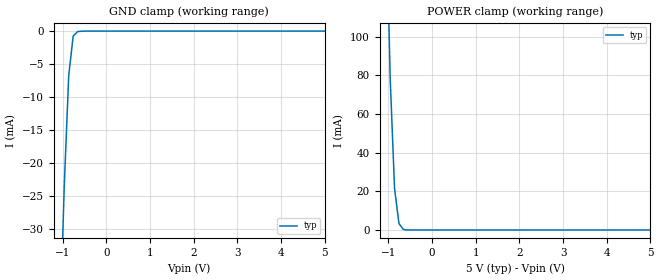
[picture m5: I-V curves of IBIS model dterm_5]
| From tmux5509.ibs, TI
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| dterm_5
[Model]   dterm_5
Model_type   Terminator
|   typ   min   max
C_comp   6.362683e-12   NA   NA
[Voltage Range]   5   NA   NA
[Temperature Range]   27   NA   NA
[Power Clamp Reference]   5   NA   NA
[GND Clamp Reference]   0   NA   NA
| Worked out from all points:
|   GND clamp passes 1 mA (typ) near -0.76 V on its own axis
|   POWER clamp passes 1 mA (typ) near -0.68 V on its own axis
[GND Clamp]
|   Voltage   I(typ)   I(min)   I(max)
-5V       -2.839A    NA         NA
-1.061V   -45mA      NA         NA
-959.6mV  -23.25mA   NA         NA
-858.6mV  -6.731mA   NA         NA
-757.6mV  -768.2uA   NA         NA
-656.6mV  -81.6uA    NA         NA
5V        469.4pA    NA         NA
[POWER Clamp]
|   Voltage   I(typ)   I(min)   I(max)
-5V       7.431A     NA         NA
-1.061V   177.8mA    NA         NA
-959.6mV  79.08mA    NA         NA
-858.6mV  21.55mA    NA         NA
-757.6mV  3.291mA    NA         NA
-656.6mV  235.7uA    NA         NA
5V        -416.2pA   NA         NA
